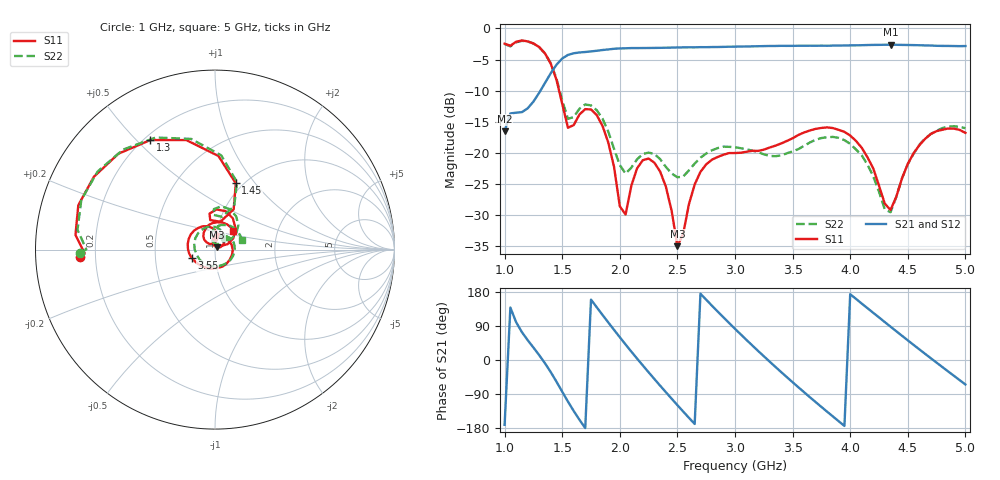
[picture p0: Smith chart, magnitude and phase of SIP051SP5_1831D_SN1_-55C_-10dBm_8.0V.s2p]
# GHz  S  dB  R  50
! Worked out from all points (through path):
!   81 points, 1 GHz to 5 GHz, reference 50 ohm
!   highest |S21| = -2.62 dB at 4.35 GHz (marker M1); lowest = -16.5 dB at 1 GHz (marker M2)
!   lowest |S11| = -35.1 dB at 2.5 GHz (marker M3), VSWR 1.04, Z = 51.2 + j1.3 ohm
!   |S11| at or under -10 dB: 1.473 GHz to end of sweep
!   |S22| runs from -29.6 to -2.0 dB; largest |S21 - S12| = 0.0022
!   S11 on the Smith chart (normalised r, x): 1 GHz: 0.14, -0.03; 1.3 GHz: 0.22, +0.55; 1.45 GHz: 0.93, +0.80; 3.55 GHz: 0.77, -0.07; 5 GHz: 1.20, +0.25
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1  -2.45 -176.8  -16.55 -171.1  -16.55 -171.0  -2.50 -178.6
1.15  -1.93 162.0  -13.49 73.7  -13.49 73.8  -2.00 159.7
1.3  -2.99 120.5  -10.37 13.0  -10.38 13.0  -3.02 117.9
1.45  -8.24 72.6  -5.85 -57.0  -5.83 -57.0  -8.06 71.9
1.55  -16.00 79.0  -4.26 -109.8  -4.26 -109.8  -14.57 78.1
1.7  -13.00 88.0  -3.79 -179.6  -3.79 -179.6  -12.25 81.8
1.85  -15.71 45.4  -3.47 118.9  -3.47 118.9  -14.53 46.1
1.95  -22.31 23.2  -3.27 79.5  -3.28 79.5  -19.42 32.8
2.05  -29.99 89.7  -3.19 41.0  -3.19 41.0  -23.39 55.1
2.15  -22.54 95.0  -3.15 3.7  -3.16 3.7  -21.08 67.7
2.35  -23.06 41.7  -3.12 -67.7  -3.11 -67.6  -21.06 43.9
2.5  -35.09 46.4  -3.06 -119.1  -3.06 -119.1  -23.98 47.6
2.7  -23.11 82.9  -3.01 175.0  -3.01 175.0  -20.83 53.2
2.85  -20.71 34.1  -2.99 127.8  -2.99 127.8  -19.28 31.4
3  -20.08 -16.5  -2.93 82.3  -2.93 82.3  -19.14 3.2
3.25  -19.53 -93.4  -2.84 10.0  -2.84 10.0  -20.29 -60.1
3.55  -17.17 -160.8  -2.79 -71.9  -2.78 -71.9  -19.44 -164.2
3.7  -16.18 168.3  -2.79 -111.0  -2.79 -111.1  -17.94 149.4
4  -17.25 108.5  -2.72 173.6  -2.73 173.6  -18.60 78.0
4.35  -29.26 114.4  -2.62 88.0  -2.62 88.0  -29.63 87.6
4.7  -17.00 104.5  -2.75 4.6  -2.75 4.6  -17.00 75.8
5  -16.82 44.8  -2.83 -64.6  -2.85 -64.7  -16.07 19.4
